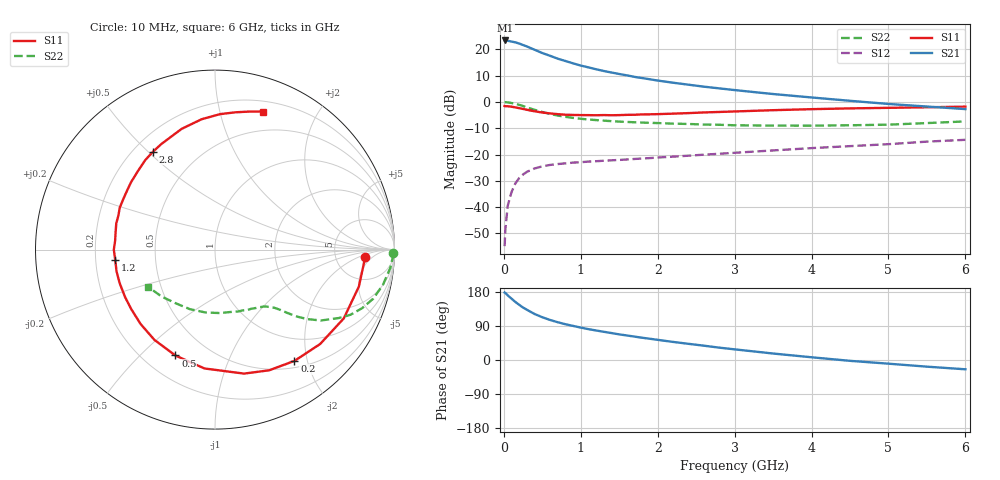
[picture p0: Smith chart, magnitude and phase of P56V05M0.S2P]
! SIEMENS Small Signal Semiconductors
! BFP183
! Si NPN RF Bipolar Junction Transistor in SOT143
! VCE = 6 V  IC = 5 mA
! Common Emitter S-Parameters:  March  1996
# GHz  S  MA  R  50
!  f  S11  S21  S12  S22
! GHz  MAG  ANG  MAG  ANG  MAG  ANG  MAG  ANG
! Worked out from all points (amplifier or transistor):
!   36 points, 10 MHz to 6 GHz, reference 50 ohm
!   highest |S21| = 23.4 dB at 20 MHz (marker M1)
!   |S21| within 3 dB of that: start of sweep to 356.9 MHz
!   unconditionally stable (mu >= 1): 1.624 GHz to 5.731 GHz
!   at 250 MHz: K = 0.20, MSG = 24.6 dB, |S12| = -27.6 dB
!   at 1.4 GHz: K = 0.92, MSG = 16.7 dB, |S12| = -22.2 dB
!   at 6 GHz: K = 0.96, MSG = 5.8 dB, |S12| = -14.4 dB
!   lowest NFmin = 1.15 dB at 450 MHz
!   S11 on the Smith chart (normalised r, x): 10 MHz: 10, -3; 200 MHz: 0.60, -1.78; 500 MHz: 0.33, -0.64; 1.2 GHz: 0.28, -0.05; 2.8 GHz: 0.28, +0.52; 6 GHz: 0.30, +1.37
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0.01  0.8371 -2.9  14.76 178.1  0.0018 85.6  0.9926 -1.2
0.02  0.8319 -6.0  14.83 176.7  0.0038 85.1  0.9915 -2.5
0.05  0.8277 -14.4  14.64 170.6  0.0105 84.7  0.9819 -6.0
0.1  0.8135 -28.1  14.12 161.9  0.0193 75.6  0.9561 -11.8
0.15  0.7874 -41.9  13.64 153.2  0.0282 68.3  0.9235 -17.2
0.2  0.7619 -54.5  12.95 145.5  0.0357 63.0  0.8825 -21.7
0.25  0.7371 -65.8  12.12 138.4  0.0417 58.1  0.8374 -25.7
0.3  0.7097 -76.8  11.41 132.5  0.0468 53.6  0.7888 -28.9
0.4  0.6648 -95.1  9.861 121.4  0.0543 46.2  0.71 -33.8
0.5  0.6298 -110.5  8.54 112.8  0.0595 41.1  0.6452 -36.9
0.6  0.6059 -123.8  7.584 105.7  0.0633 37.8  0.5931 -39.1
0.7  0.5864 -134.9  6.676 99.7  0.0658 35.3  0.5517 -40.6
0.9  0.5665 -152.3  5.435 90.0  0.0701 32.1  0.498 -42.6
1.1  0.5619 -167.6  4.556 81.4  0.0734 30.6  0.4633 -44.4
1.2  0.5587 -174.1  4.191 77.9  0.0745 29.8  0.4524 -45.4
1.7  0.5709 160.5  3.004 61.7  0.0823 30.3  0.4108 -51.1
2.2  0.5998 141.3  2.327 47.7  0.0911 30.9  0.3867 -58.5
2.8  0.6458 122.3  1.816 32.6  0.1033 30.9  0.368 -69.7
3.5  0.698 105.4  1.417 17.1  0.1196 30.2  0.3548 -85.4
4.5  0.7552 87.9  1.053 -2.2  0.1444 26.3  0.3601 -112.9
5.5  0.7929 75.9  0.819 -17.6  0.176 21.9  0.3966 -138.9
6  0.8149 70.7  0.732 -24.5  0.1904 18.1  0.4269 -151.0
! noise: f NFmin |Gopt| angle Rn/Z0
0.45  1.15  0.25  40  0.26
0.9  1.2  0.25  93  0.22
1.8  1.95  0.32  170  0.13
